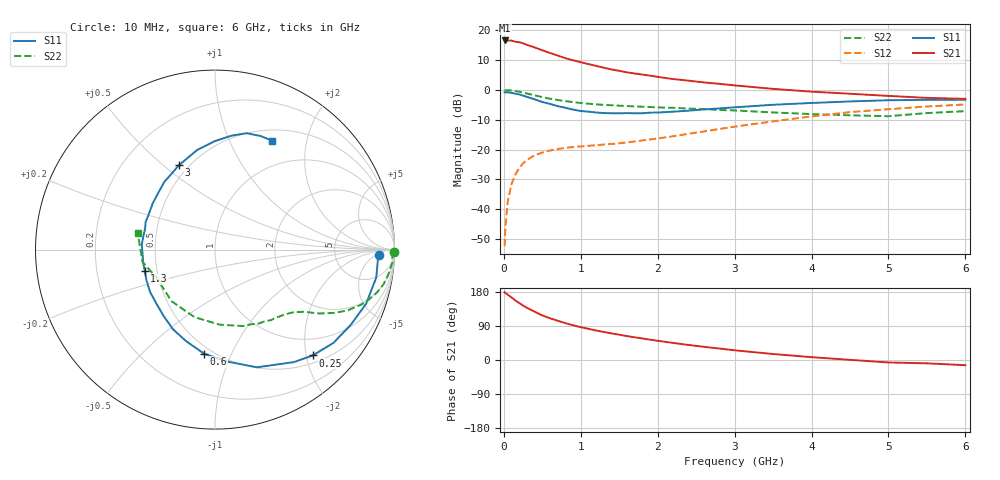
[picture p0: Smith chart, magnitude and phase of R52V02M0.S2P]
! SIEMENS Small Signal Semiconductors
! BFR183
! Si NPN RF Bipolar Junction Transistor in SOT23
! VCE = 2 V  IC = 2 mA
! Common Emitter S-Parameters:  May  1996
# GHz  S  MA  R  50
!  f  S11  S21  S12  S22
! GHz  MAG  ANG  MAG  ANG  MAG  ANG  MAG  ANG
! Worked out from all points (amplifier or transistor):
!   36 points, 10 MHz to 6 GHz, reference 50 ohm
!   highest |S21| = 16.6 dB at 10 MHz (marker M1)
!   |S21| within 3 dB of that: start of sweep to 469.4 MHz
!   unconditionally stable (mu >= 1): 1.369 GHz to 2.846 GHz
!   at 250 MHz: K = 0.23, MSG = 20.1 dB, |S12| = -24.6 dB
!   at 1.4 GHz: K = 1.01, MAG = 11.8 dB, |S12| = -18.1 dB
!   at 6 GHz: K = 0.92, MSG = 0.9 dB, |S12| = -4.9 dB
!   S11 on the Smith chart (normalised r, x): 10 MHz: 19, -7; 250 MHz: 0.64, -2.12; 600 MHz: 0.45, -0.79; 1.3 GHz: 0.43, -0.12; 3 GHz: 0.44, +0.56; 6 GHz: 0.64, +1.45
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0.01  0.9131 -2.0  6.755 178.9  0.0024 89.9  0.9963 -0.8
0.02  0.909 -4.1  6.632 176.9  0.005 93.4  0.9876 -1.6
0.05  0.9119 -9.8  6.725 172.5  0.0133 85.2  0.9914 -4.0
0.1  0.8943 -19.7  6.71 165.1  0.0264 79.2  0.9764 -8.0
0.15  0.8651 -28.9  6.423 157.1  0.0382 74.0  0.9584 -11.7
0.2  0.8401 -38.2  6.313 150.3  0.049 69.1  0.9329 -14.9
0.25  0.8026 -47.3  6.058 143.6  0.0588 64.5  0.9005 -18.1
0.3  0.7653 -55.0  5.691 137.7  0.0669 61.0  0.8709 -20.6
0.4  0.696 -70.4  5.163 127.5  0.0802 54.7  0.8132 -24.6
0.5  0.6276 -83.7  4.623 117.7  0.0892 49.9  0.7568 -27.7
0.6  0.5833 -95.9  4.164 110.1  0.0965 46.5  0.7118 -29.9
0.8  0.5019 -117.8  3.413 97.3  0.1067 42.3  0.6483 -32.9
0.9  0.4676 -127.8  3.141 91.6  0.1105 41.6  0.6249 -33.9
1.1  0.4319 -146.9  2.715 82.2  0.1156 41.8  0.5873 -36.3
1.3  0.4095 -162.8  2.356 74.0  0.1216 42.7  0.561 -38.2
1.6  0.409 176.0  1.97 63.1  0.1318 45.4  0.5366 -42.0
2.2  0.4322 143.4  1.522 45.1  0.167 51.7  0.5022 -51.4
3  0.511 113.3  1.192 25.6  0.2424 52.5  0.4534 -70.0
3.5  0.564 100.1  1.042 15.8  0.297 48.9  0.4192 -86.3
4.5  0.6412 81.8  0.863 0.4  0.4247 36.8  0.376 -130.1
5.5  0.6819 68.1  0.736 -8.8  0.5273 22.3  0.4095 -170.3
6  0.685 62.4  0.709 -13.7  0.5704 13.1  0.4408 167.7
